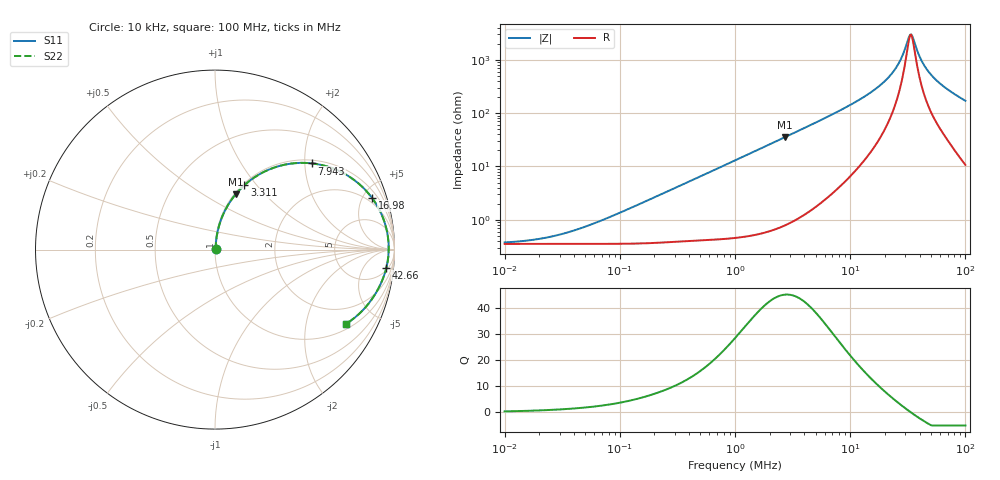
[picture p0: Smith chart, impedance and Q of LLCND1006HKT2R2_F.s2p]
! LLCND1006HKT2R2_F  S-PARAMETER MODEL  ( Standard Model )
! Model Generated by TAIYO YUDEN Corporation (http://www.ty-top.com)
! Version 2.0
! TAIYO YUDEN Control No. 231226
! Copyright(c) 2023 TAIYO YUDEN CO.,LTD. All Rights Reserved.
! Product Description (link to TY-COMPAS)
! https://ds.yuden.co.jp/TYCOMPAS/or/detail?pn=LLCND1006HKT2R2MF&u=M
! Products Name : Inductors
! Characteristics :
!  Inductance : 2.2 [uH] , SRF(min) : - [Hz] , DC Resistance(max) : 375 [mOhm]
!  Rated Current : Saturation  0.8 [A] (dL = 30 [%]), Temp Rise  0.6 [A] (dT = 40 [degC])
!  Case Size : 1.0 x 0.6 / 0.039 x 0.024 [mm/inch] , Thickness : 0.8 / 0.031 [mm/inch]
!  (Conditions: Temperature = 25 [degC] , DC Bias Current = 0 [A])
! External Node Assignments :
!  1  o---GGG---o  2
! GND o---------o GND
! Frequency Range : 10kHz  -  100MHz  [ 402 STEP ]
# MHz S RI R 50
! Freq[MHz].  S11 Real  S11 Imag  S21 Real  S21 Imag  S12 Real  S12 Imag  S22 Real  S22 Imag
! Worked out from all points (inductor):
!   401 points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, 10 kHz to 100 MHz, reference 50 ohm
!   read as one part in series: L = 2.09 uH near 83.18 kHz
!   highest Q = 44.9 at 2.692 MHz (marker M1), where L = 2.07 uH
!   self-resonance near 33.62 MHz
!   S11 on the Smith chart (normalised r, x): 10 kHz: 1.01, +0.00; 3.311 MHz: 1.02, +0.87; 7.943 MHz: 1.08, +2.18; 16.98 MHz: 1.54, +5.86; 42.66 MHz: 6, -17; 100 MHz: 1.21, -3.39
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0.01  0.00353 0.0013  0.9965 -0.0013  0.9965 -0.0013  0.00353 0.0013
0.022387  0.00354 0.00291  0.9965 -0.00291  0.9965 -0.00291  0.00354 0.00291
0.046774  0.00357 0.00608  0.9964 -0.00608  0.9964 -0.00608  0.00357 0.00608
0.218776  0.00453 0.0284  0.9955 -0.0284  0.9955 -0.0284  0.00453 0.0284
1  0.0209 0.1264  0.9791 -0.1264  0.9791 -0.1264  0.0209 0.1264
2.691535  0.115 0.308  0.885 -0.308  0.885 -0.308  0.115 0.308
3.311311  0.1634 0.3587  0.8366 -0.3587  0.8366 -0.3587  0.1634 0.3587
4.677351  0.2811 0.437  0.7189 -0.437  0.7189 -0.437  0.2811 0.437
7.943282  0.541 0.4803  0.459 -0.4803  0.459 -0.4803  0.541 0.4803
12.02264  0.7487 0.4063  0.2513 -0.4063  0.2513 -0.4063  0.7487 0.4063
16.98244  0.8753 0.2872  0.1247 -0.2872  0.1247 -0.2872  0.8753 0.2872
21.87762  0.9332 0.1839  0.0668 -0.1839  0.0668 -0.1839  0.9332 0.1839
26.91535  0.9593 0.0956  0.0407 -0.0956  0.0407 -0.0956  0.9593 0.0956
31.62278  0.9673 0.0263  0.0327 -0.0263  0.0327 -0.0263  0.9673 0.0263
33.11311  0.9677 0.00655  0.0323 -0.00655  0.0323 -0.00655  0.9677 0.00655
34.67368  0.9672 -0.0132  0.0328 0.0132  0.0328 0.0132  0.9672 -0.0132
39.81072  0.9608 -0.0718  0.0392 0.0718  0.0392 0.0718  0.9608 -0.0718
42.65795  0.9548 -0.1008  0.0452 0.1008  0.0452 0.1008  0.9548 -0.1008
48.97788  0.9373 -0.1575  0.0627 0.1575  0.0627 0.1575  0.9373 -0.1575
58.88437  0.9032 -0.2301  0.0968 0.2301  0.0968 0.2301  0.9032 -0.2301
75.85776  0.836 -0.3243  0.164 0.3243  0.164 0.3243  0.836 -0.3243
100  0.7302 -0.4134  0.2698 0.4134  0.2698 0.4134  0.7302 -0.4134
